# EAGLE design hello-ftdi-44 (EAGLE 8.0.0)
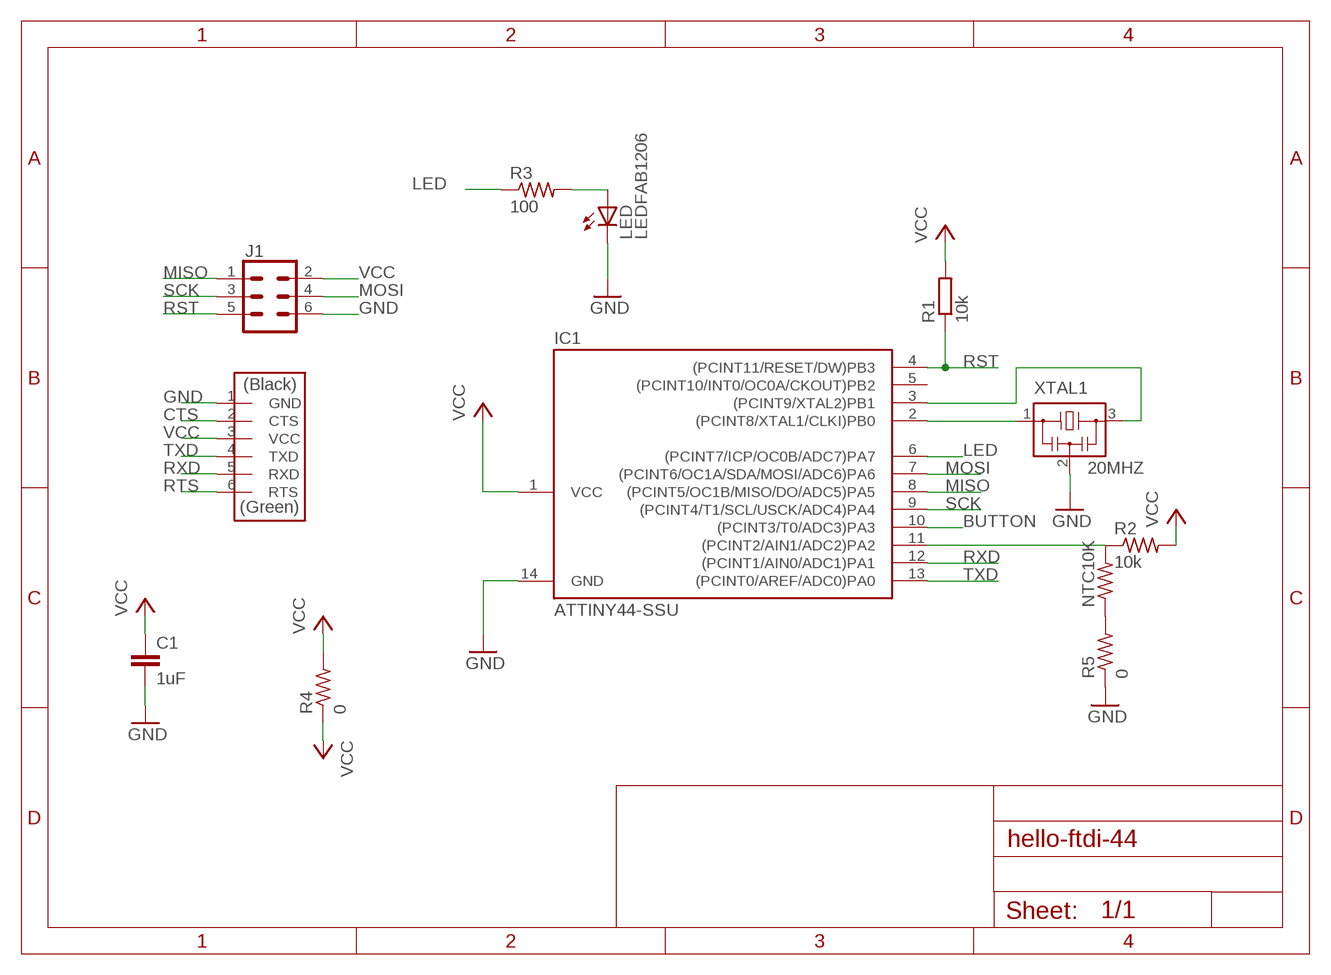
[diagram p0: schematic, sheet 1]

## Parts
C1  1uF  C-EUC1206  [C1206]
IC1  ATTINY44-SSU  [SOIC14]
J1  CONN_03X2SMT  [2X3_SMT_POSTS]
J2  FTDI-SMD-HEADER  [1X06SMD]
LED  LEDFAB1206  [LED1206FAB]
NTC10K  RES-US1206  [R1206]
R1  10k  R-EU_M1206  [M1206]
R2  10k  RES-US1206  [R1206]
R3  100  RES-US1206  [R1206]
R4  0  RES-US1206FAB  [R1206FAB]
R5  0  RES-US1206FAB  [R1206FAB]
XTAL1  20MHZ  RESONATOR  [EFOBM]

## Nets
BUTTON: IC1.10((PCINT3/T0/ADC3)PA3)
CTS: J2.2(CTS)
GND: C1.2 IC1.14(GND) J1.6 J2.1(GND) LED.2(C) R5.1 XTAL1.2
LED: IC1.6((PCINT7/ICP/OC0B/ADC7)PA7) R3.1
MISO: IC1.8((PCINT5/OC1B/MISO/DO/ADC5)PA5) J1.1
MOSI: IC1.7((PCINT6/OC1A/SDA/MOSI/ADC6)PA6) J1.4
N$1: IC1.11((PCINT2/AIN1/ADC2)PA2) NTC10K.2 R2.1
N$2: LED.1(A) R3.2
N$3: NTC10K.1 R5.2
N$7: IC1.2((PCINT8/XTAL1/CLKI)PB0) XTAL1.1
N$8: IC1.3((PCINT9/XTAL2)PB1) XTAL1.3
RST: IC1.4((PCINT11/RESET/DW)PB3) J1.5 R1.1
RTS: J2.6(RTS)
RXD: IC1.12((PCINT1/AIN0/ADC1)PA1) J2.5(RXD)
SCK: IC1.9((PCINT4/T1/SCL/USCK/ADC4)PA4) J1.3
TXD: IC1.13((PCINT0/AREF/ADC0)PA0) J2.4(TXD)
VCC: C1.1 IC1.1(VCC) J1.2 J2.3(VCC) R1.2 R2.2 R4.1 R4.2
Unconnected: IC1.5((PCINT10/INT0/OC0A/CKOUT)PB2)

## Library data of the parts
C1 = rcl:C-EU: CAPACITOR, European symbol
IC1 = fab:ATTINY44
J1 = SparkFun-Connectors:CONN_03X2: Multi connection point. Often used as Generic Header-pin footprint for 0.1 inch spaced/style header connections You can populate with any combo of single row headers, but if you'd like an exact match, check these: Header - 2x3 (Male, 0.1") (PRT-12807) Header - 2x3 (Female, 0.1") (PRT-13010) 2x3 Pin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; PROD_ID: CONN-11415
J2 = fab:FTDI-SMD-HEADER
LED = fab:LED: LED
NTC10K R2-R5 = fab:RES-US: Resistor (US Symbol)
R1 = rcl:R-EU_: RESISTOR, European symbol
XTAL1 = fab:RESONATOR

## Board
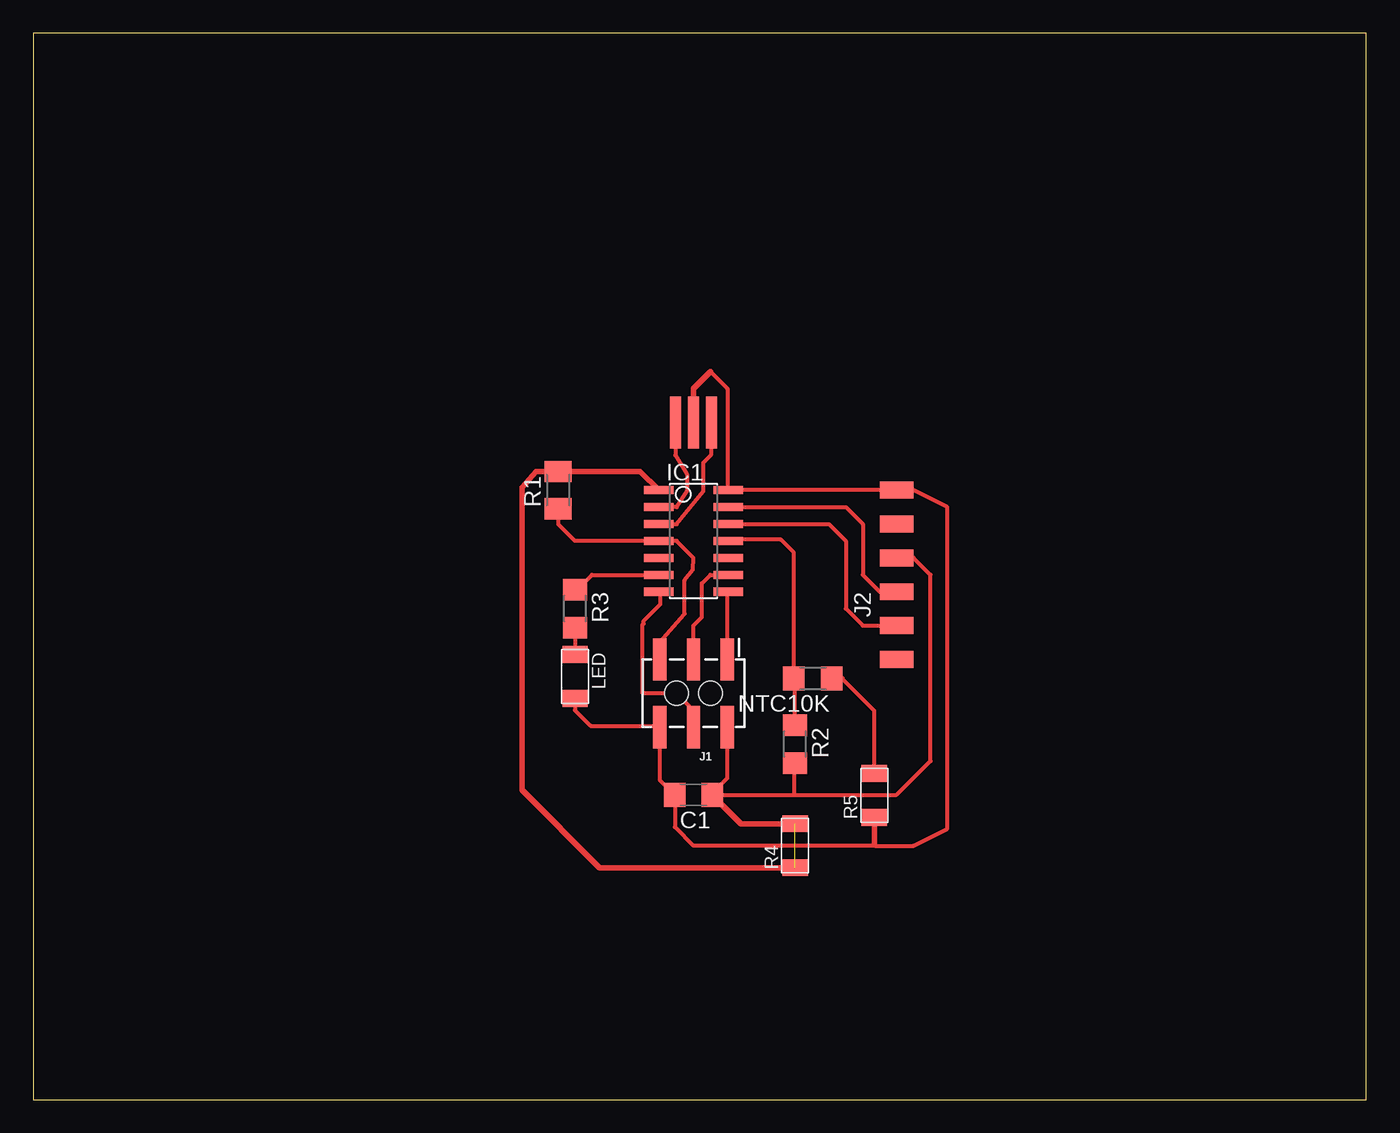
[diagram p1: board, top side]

Size 100 x 80 mm. Coordinates in mm from the lower left corner, seen from the top.
Outline: 0,0 100,0 100,80 0,80 0,0
Copper layers (1*16): Top 0.035mm / dielectric 1.5mm / Bottom 0.035mm
Design rules "default *": minimum track width 12mil, minimum drill 16mil, track to track 16mil, track to pad 16mil, pad to pad 16mil, via to via 16mil, smd to smd 16mil, copper to edge 16mil, drill to drill 16mil, minimum pad ring 10mil, minimum via ring 8mil, stop-mask expansion 4mil, vias tented up to drill 0mil, thermal gap 10mil

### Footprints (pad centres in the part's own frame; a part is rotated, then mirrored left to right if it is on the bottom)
C1206 = smd 1.6 x 1.8: 1 -1.4,0; 2 1.4,0
SOIC14 = smd 0.61 x 2.21: 1 -3.81,-2.603; 2 -2.54,-2.603; 3 -1.27,-2.603; 4 0,-2.603; 5 1.27,-2.603; 6 2.54,-2.603; 7 3.81,-2.603; 8 3.81,2.603; 9 2.54,2.603; 10 1.27,2.603; 11 0,2.603; 12 -1.27,2.603; 13 -2.54,2.603; 14 -3.81,2.603
2X3_SMT_POSTS = smd 1 x 3.17: 1 -2.54,-2.54; 2 -2.54,2.54; 3 0,-2.54; 4 0,2.54; 5 2.54,-2.54; 6 2.54,2.54 | hole 1.8: -1.27,0; 1.27,0
1X06SMD = smd 2.54 x 1.27: 1 0,6.35; 2 0,3.81; 3 0,1.27; 4 0,-1.27; 5 0,-3.81; 6 0,-6.35
LED1206FAB = smd 1.27 x 1.905: 1 -1.651,0; 2 1.651,0
R1206 = smd 1.6 x 1.803: 1 -1.422,0; 2 1.422,0
M1206 = smd 1.6 x 2: 1 -1.4,0; 2 1.4,0
R1206FAB = smd 1.27 x 1.905: 1 -1.651,0; 2 1.651,0
EFOBM = smd 0.8 x 3.9: 1 -1.35,0; 2 0,0; 3 1.35,0

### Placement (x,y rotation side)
C1  49.53,22.86 180 top
IC1  49.53,41.91 270 top
J1  49.53,30.48 180 top
J2  64.77,39.37 0 top
LED  40.64,31.75 270 top
NTC10K  58.48,31.6 180 top
R1  39.37,45.72 90 top
R2  57.15,26.67 270 top
R3  40.64,36.83 270 top
R4  57.15,19.05 90 top
R5  63.09,22.82 90 top
XTAL1  49.53,50.8 0 top

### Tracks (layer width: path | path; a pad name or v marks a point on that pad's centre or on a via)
GND
  Top 0.305: LED.2 40.64,29.21 41.81,28.04 46.89,28.04 J1.6 46.99,24 C1.2 48.13,20.45 49.53,19.05 63.13,19.05 | 50.8,54.61 52.07,53.34 52.07,45.78 IC1.14 J2.1 66.04,45.72 68.58,44.45 68.58,20.32 66.04,19.05 63.13,19.05 | 63.09,19.21 63.09,19.08 63.13,19.05
  Top 0.406: XTAL1.2 49.53,53.34 50.8,54.61 | 46.89,28.04 J1.6 | R5.1 63.09,19.21
LED
  Top 0.305: R3.1 40.79,38.25 41.91,39.37 IC1.6
MISO
  Top 0.305: J1.1 52.07,38.04 IC1.8
MOSI
  Top 0.305: J1.4 49.53,29.21 48.26,30.48 45.72,30.48 45.72,35.65 45.79,35.71 45.79,35.91 47.04,37.16 47.04,37.99 IC1.7
  Top 0.406: IC1.7 47.01,38.01
N$1
  Top 0.305: R2.1 57.15,31.51 NTC10K.2 57.06,41.03 56.08,42.01 52.23,42.01 IC1.11
  Top 0.406: 57.08,31.62 NTC10K.2 | 57.06,28.18 R2.1
N$2
  Top 0.305: R3.2 LED.1
N$3
  Top 0.305: R5.2 63.09,29.16 60.65,31.6
  Top 0.406: 60.65,31.6 NTC10K.1 | 63.04,24.52 R5.2
N$7
  Top 0.305: XTAL1.1 48.18,48.34 49.04,46.93 49.04,45.66 48.26,44.45 IC1.2
N$8
  Top 0.305: IC1.3 48.26,43.18 50.27,45.65 50.27,47.79 50.88,48.4 XTAL1.3
RST
  Top 0.305: R1.1 39.37,43.18 40.64,41.91 IC1.4 48.26,41.91 49.53,40.64 49.49,39.76 48.86,38.98 48.86,36.44 46.99,34.29 J1.5
RXD
  Top 0.305: IC1.12 59.69,43.18 60.96,41.91 60.96,36.83 62.23,35.56 J2.5
SCK
  Top 0.305: J1.3 49.53,35.56 50.16,36.2 50.16,38.73 50.8,39.37 IC1.9
TXD
  Top 0.305: IC1.13 60.96,44.45 62.23,43.18 62.23,39.37 63.5,38.1 J2.4
VCC  (1 unrouted)
  Top 0.305: J1.2 52.07,24.13 50.93,22.99 C1.1 57.1,22.86 | 57.1,22.86 64.77,22.86 67.31,25.4 67.31,39.37 66.04,40.64 J2.3 | 57.1,22.86 57.1,25.2 R2.2
  Top 0.406: IC1.1 45.53,47.12 R1.2 39.24,47.11 37.73,47.11 36.65,45.91 36.65,23.24 42.49,17.4 R4.1 | C1.1 53.09,20.7 R4.2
